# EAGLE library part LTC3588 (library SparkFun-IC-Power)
Energy Harvesting Power Supply(IC-09818)
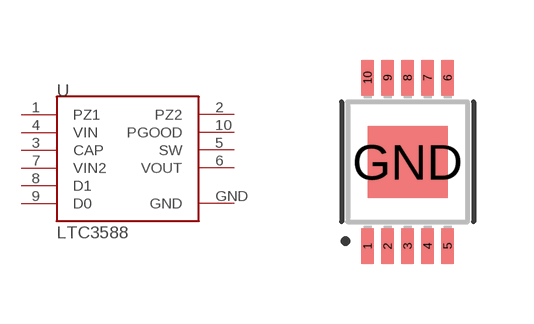
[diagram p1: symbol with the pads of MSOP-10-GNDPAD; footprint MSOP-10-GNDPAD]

Designator prefix U

## LTC3588_  [MSOP-10-GNDPAD]
1  PZ1
2  PZ2
3  CAP
4  VIN
5  SW
6  VOUT
7  VIN2
8  D1
9  D0
10  PGOOD
GND  GND

## Footprint MSOP-10-GNDPAD (pad centres in mm)
10-lead MSOP w/ center GND pad
smd 0.305 x 0.889: 1 -1,-2.11; 2 -0.5,-2.11; 3 0,-2.11; 4 0.5,-2.11; 5 1,-2.11; 6 1,2.11; 7 0.5,2.11; 8 0,2.11; 9 -0.5,2.11; 10 -1,2.11
smd 2 x 1.8: GND 0,0

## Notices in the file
Licensing: Creative Commons ShareAlike 4.0 International - https://creativecommons.org/licenses/by-sa/4.0
